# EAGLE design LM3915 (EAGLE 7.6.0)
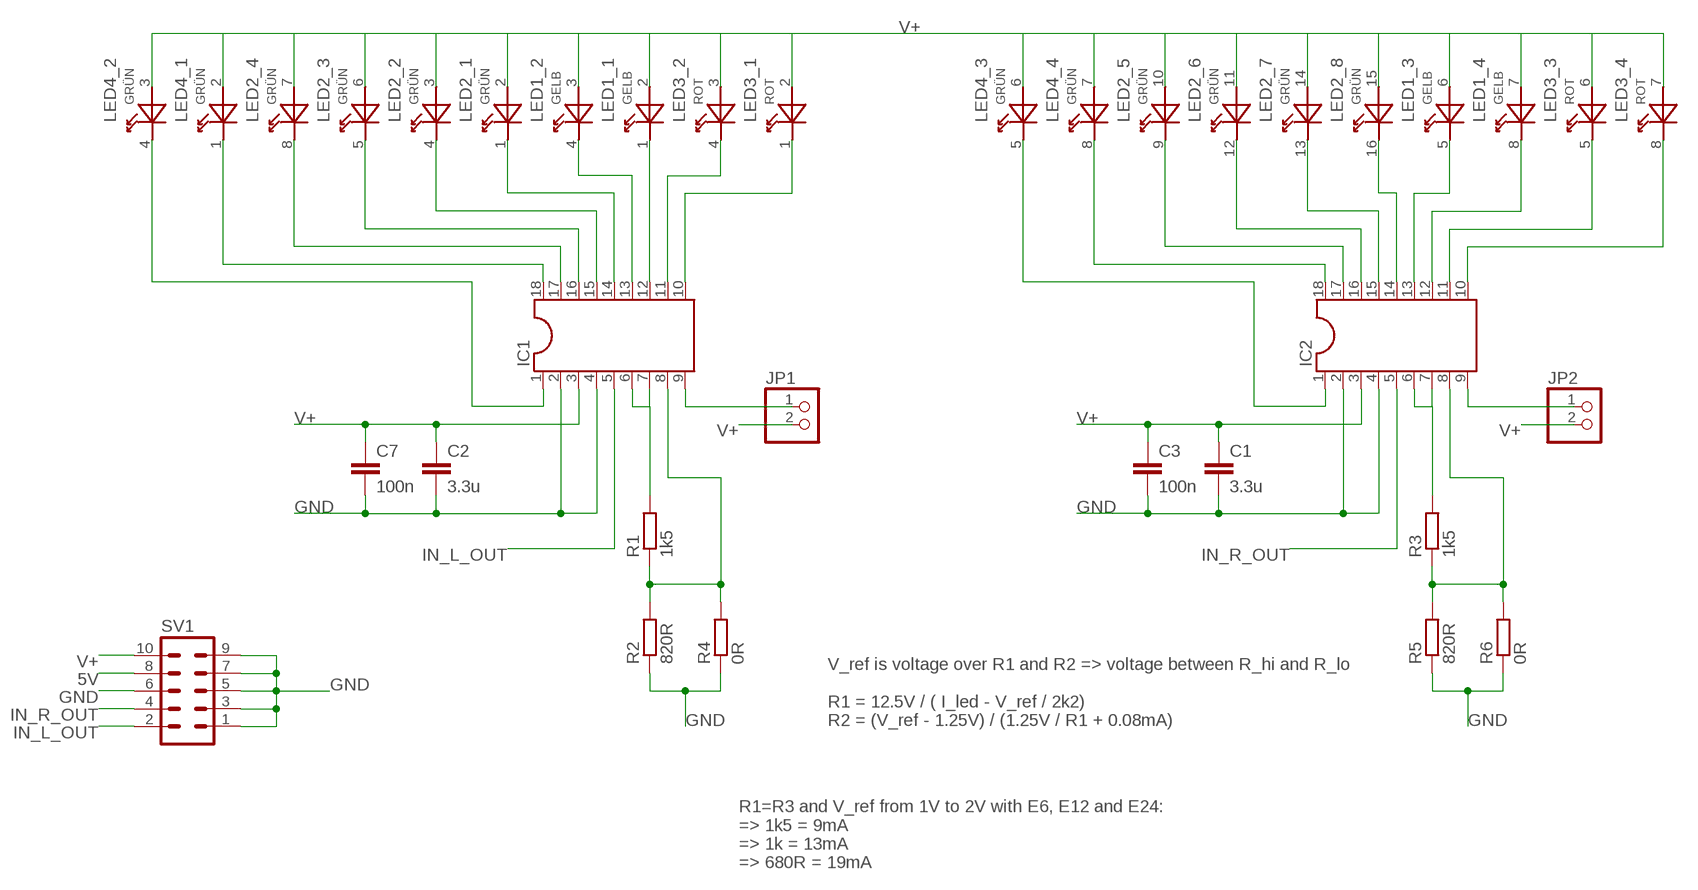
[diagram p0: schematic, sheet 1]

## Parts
C1  3.3u  C-EU050-055X075  [C050-055X075]
C2  3.3u  C-EU050-055X075  [C050-055X075]
C3  100n  C-EU050-025X075  [C050-025X075]
C7  100n  C-EU050-025X075  [C050-025X075]
IC1  DIL18S  [SOCKET-18]
IC2  DIL18S  [SOCKET-18]
JP1  PINHD-1X2  [1X02]
JP2  PINHD-1X2  [1X02]
LED1  GELB  KB-27XX-2  [KB-27XX]
LED2  GRÜN  KB-28XX-4  [KB-28XX]
LED3  ROT  KB-27XX-2  [KB-27XX]
LED4  GRÜN  KB-27XX-2  [KB-27XX]
R1  1k5  R-EU_0309/V  [0309V]
R2  820R  R-EU_0309/V  [0309V]
R3  1k5  R-EU_0309/V  [0309V]
R4  0R  R-EU_R0603  [R0603]
R5  820R  R-EU_0309/V  [0309V]
R6  0R  R-EU_R0603  [R0603]
SV1  ML10  [ML10]

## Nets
5V: SV1.8
GND: C1.2 C2.2 C3.2 C7.2 IC1.2 IC1.4 IC2.2 IC2.4 R2.1 R4.1 R5.1 R6.1 SV1.1 SV1.3 SV1.5 SV1.6 SV1.7 SV1.9
IN_L_OUT: IC1.5 SV1.2
IN_R_OUT: IC2.5 SV1.4
N$1: IC1.9 JP1.1
N$2: IC1.6 IC1.7 R1.2
N$3: IC1.8 R1.1 R2.2 R4.2
N$4: IC2.6 IC2.7 R3.2
N$5: IC2.9 JP2.1
N$6: IC2.8 R3.1 R5.2 R6.2
N$7: IC1.1 LED4.4(_2:P1)
N$8: IC1.18 LED4.1(_1:P1)
N$9: IC1.17 LED2.8(_4:P1)
N$10: IC1.16 LED2.5(_3:P1)
N$11: IC1.15 LED2.4(_2:P1)
N$12: IC1.14 LED2.1(_1:P1)
N$13: IC1.13 LED1.4(_2:P1)
N$14: IC1.12 LED1.1(_1:P1)
N$15: IC1.11 LED3.4(_2:P1)
N$16: IC1.10 LED3.1(_1:P1)
N$18: IC2.18 LED4.8(_4:P1)
N$19: IC2.17 LED2.9(_5:P1)
N$20: IC2.16 LED2.12(_6:P1)
N$21: IC2.15 LED2.13(_7:P1)
N$22: IC2.14 LED2.16(_8:P1)
N$23: IC2.13 LED1.5(_3:P1)
N$24: IC2.12 LED1.8(_4:P1)
N$25: IC2.11 LED3.5(_3:P1)
N$26: IC2.10 LED3.8(_4:P1)
N$27: IC2.1 LED4.5(_3:P1)
V+: C1.1 C2.1 C3.1 C7.1 IC1.3 IC2.3 JP1.2 JP2.2 LED1.2(_1:P2) LED1.3(_2:P2) LED1.6(_3:P2) LED1.7(_4:P2) LED2.2(_1:P2) LED2.3(_2:P2) LED2.6(_3:P2) LED2.7(_4:P2) LED2.10(_5:P2) LED2.11(_6:P2) LED2.14(_7:P2) LED2.15(_8:P2) LED3.2(_1:P2) LED3.3(_2:P2) LED3.6(_3:P2) LED3.7(_4:P2) LED4.2(_1:P2) LED4.3(_2:P2) LED4.6(_3:P2) LED4.7(_4:P2) SV1.10

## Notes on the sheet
- V_ref is voltage over R1 and R2 => voltage between R_hi and R_lo
  
  R1 = 12.5V / ( I_led - V_ref / 2k2)
  R2 = (V_ref - 1.25V) / (1.25V / R1 + 0.08mA)
- R1=R3 and V_ref from 1V to 2V with E6, E12 and E24:
  => 1k5 = 9mA 
  => 1k = 13mA
  => 680R = 19mA

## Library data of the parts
C1-C3 C7 = rcl:C-EU: CAPACITOR, European symbol
IC1 IC2 = ic-package:DIL18: Dual In Line / Socket
JP1 JP2 = pinhead:PINHD-1X2: PIN HEADER
LED1 LED3 LED4 = my:KB-27XX-2: FW-LED 10x10 GE reichelt.de
LED2 = my:KB-28XX-4: FW-LED 10X20 GN reichelt.de
R1-R6 = rcl:R-EU_: RESISTOR, European symbol
SV1 = con-ml:ML10: HARTING; OC_FARNELL: unknown; OC_NEWARK: unknown

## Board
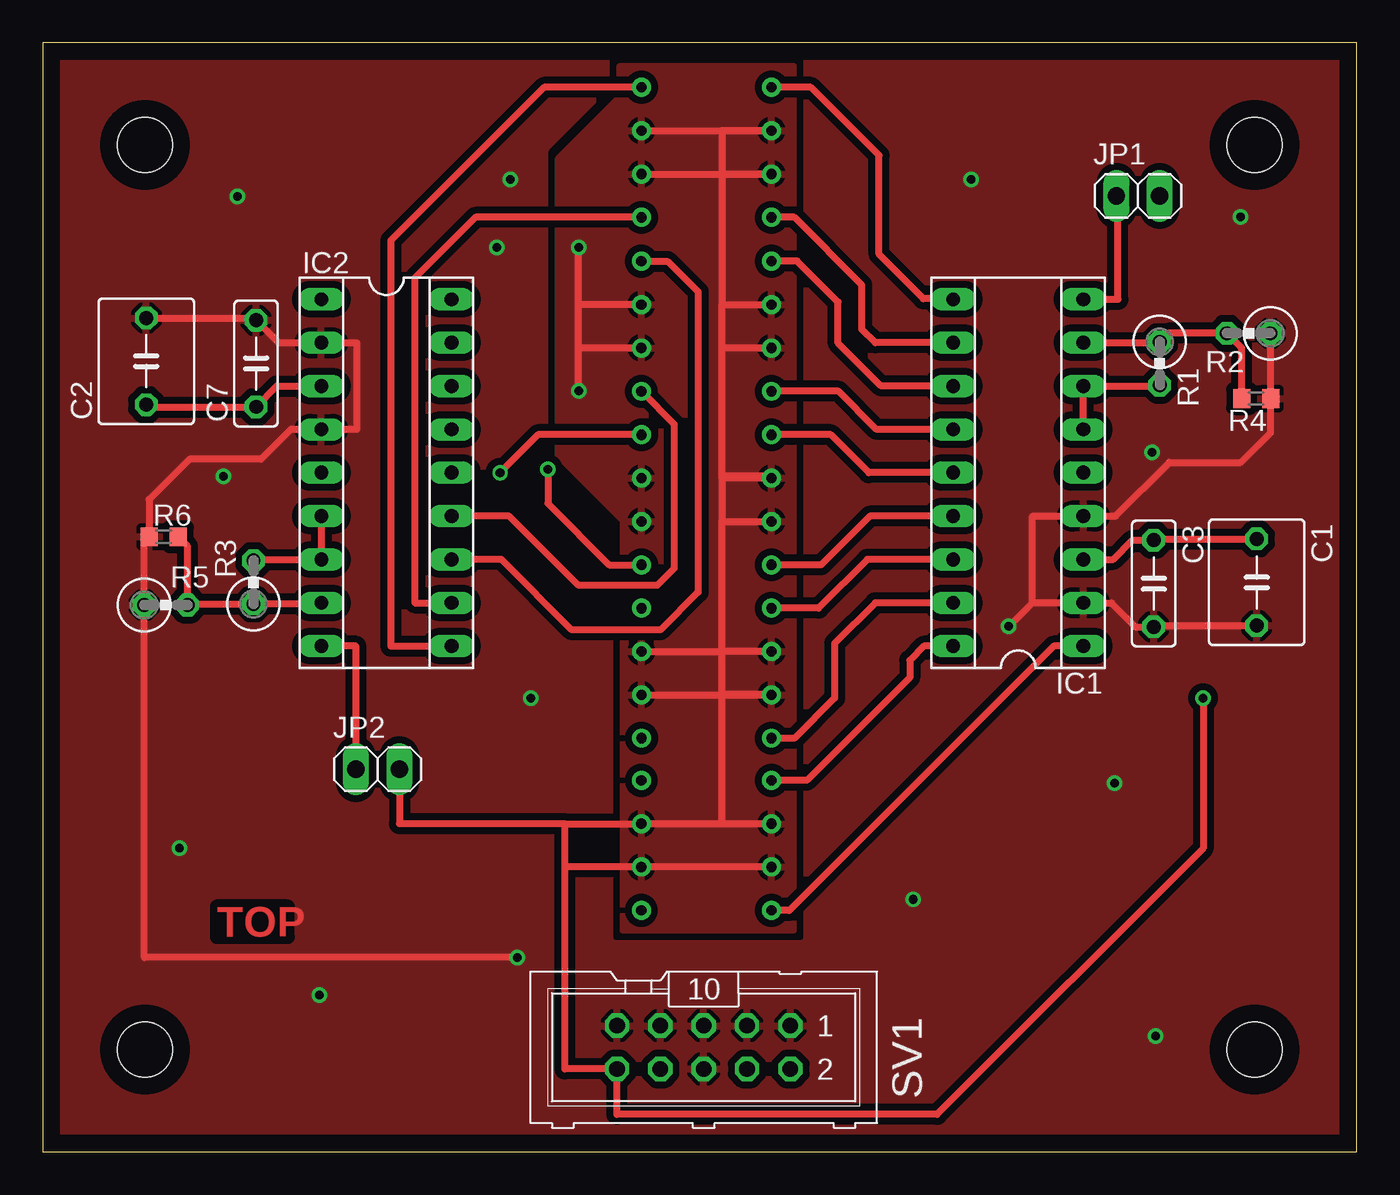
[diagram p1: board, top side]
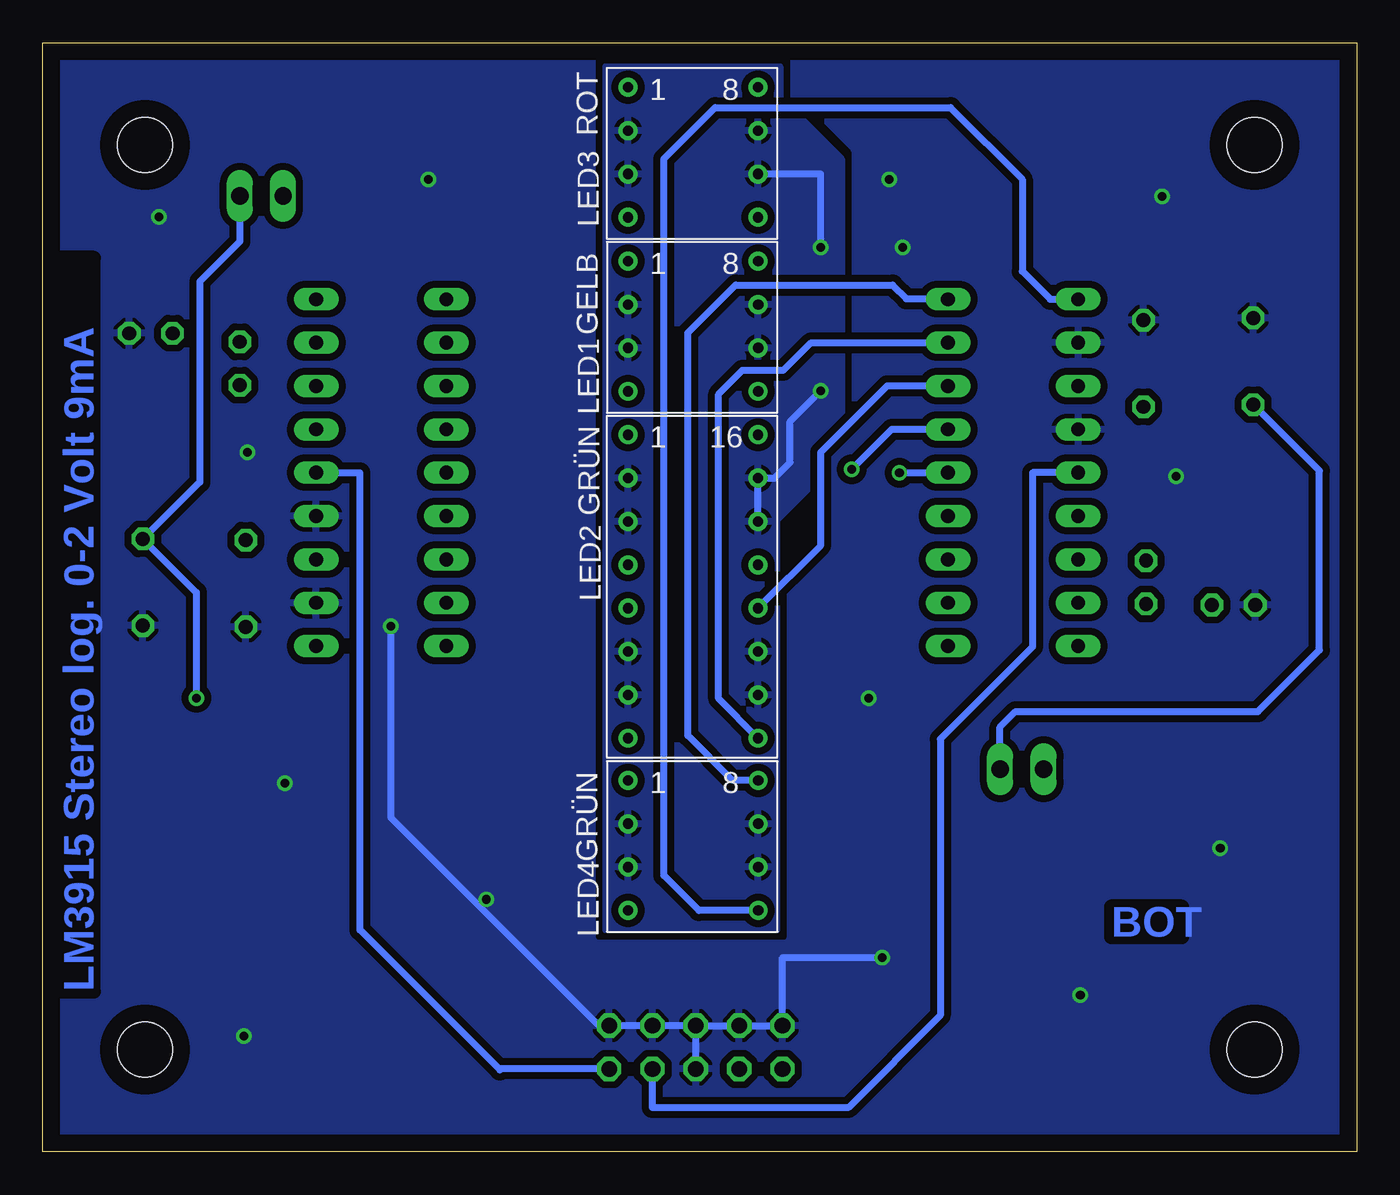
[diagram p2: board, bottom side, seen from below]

Size 77 x 65 mm. Coordinates in mm from the lower left corner, seen from the top.
Outline: 0,0 77,0 77,65 0,65 0,0
Copper layers (1*16): Top 0.035mm / dielectric 1.5mm / Bottom 0.035mm
Design rules "default *": minimum track width 10mil, minimum drill 0.5mm, track to track 8mil, track to pad 8mil, pad to pad 8mil, via to via 8mil, smd to smd 8mil, copper to edge 40mil, drill to drill 8mil, minimum pad ring 10mil, minimum via ring 8mil, stop-mask expansion 4mil, vias tented up to drill 0mil, thermal gap 10mil
Holes 3.2 mm at 6,59 6,6 71,59 71,6

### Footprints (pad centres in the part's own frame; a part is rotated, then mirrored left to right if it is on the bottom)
C050-055X075 = drill 0.813 octagon: 1 -2.54,0; 2 2.54,0
C050-025X075 = drill 0.813 octagon: 1 -2.54,0; 2 2.54,0
SOCKET-18 = drill 0.813 long: 1 -10.16,-3.81; 2 -7.62,-3.81; 3 -5.08,-3.81; 4 -2.54,-3.81; 5 0,-3.81; 6 2.54,-3.81; 7 5.08,-3.81; 8 7.62,-3.81; 9 10.16,-3.81; 10 10.16,3.81; 11 7.62,3.81; 12 5.08,3.81; 13 2.54,3.81; 14 0,3.81; 15 -2.54,3.81; 16 -5.08,3.81; 17 -7.62,3.81; 18 -10.16,3.81
1X02 = drill 1.016 long: 1 -1.27,0; 2 1.27,0
KB-27XX = drill 0.6: 1 0,0; 2 0,-2.54; 3 0,-5.08; 4 0,-7.62; 5 7.62,-7.62; 6 7.62,-5.08; 7 7.62,-2.54; 8 7.62,0
KB-28XX = drill 0.6: 1 0,0; 2 0,-2.54; 3 0,-5.08; 4 0,-7.62; 5 0,-10.16; 6 0,-12.7; 7 0,-15.24; 8 0,-17.78; 9 7.62,-17.78; 10 7.62,-15.24; 11 7.62,-12.7; 12 7.62,-10.16; 13 7.62,-7.62; 14 7.62,-5.08; 15 7.62,-2.54; 16 7.62,0
0309V = drill 0.813 octagon: 1 -1.27,0; 2 1.27,0
R0603 = smd 1 x 1.1: 1 -0.85,0; 2 0.85,0
ML10 = drill 0.914 octagon: 1 -5.08,-1.27; 2 -5.08,1.27; 3 -2.54,-1.27; 4 -2.54,1.27; 5 0,-1.27; 6 0,1.27; 7 2.54,-1.27; 8 2.54,1.27; 9 5.08,-1.27; 10 5.08,1.27

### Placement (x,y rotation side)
C1  71.13,33.38 270 top
C2  6.07,46.33 90 top
C3  65.1,33.31 270 top
C7  12.5,46.2 90 top
IC1  57.16,39.8 90 top
IC2  20.14,39.8 270 top
JP1  64.18,56.03 0 top
JP2  19.63,22.43 0 top
LED1  42.7,52.19 0 bottom
LED2  42.7,42.02 0 bottom
LED3  42.7,62.38 0 bottom
LED4  42.7,21.77 0 bottom
R1  65.45,46.2 270 top
R2  70.66,47.97 180 top
R3  12.35,33.38 90 top
R4  71.1,44.15 180 top
R5  7.22,32.05 0 top
R6  7.09,36.05 0 top
SV1  38.73,6.13 180 top

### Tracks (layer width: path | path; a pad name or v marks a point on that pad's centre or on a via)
GND  (via drill 0.5)
  Top 0.406: C2.2 12.5,48.87 C7.2 13.82,47.42 IC2.2 18.4,47.42 18.4,42.34 IC2.4 14.54,42.34 12.8,40.6 8.6,40.6 6.24,38.24 R6.1 5.95,35.76 R5.1 5.95,11.4 v27.8,11.4 | R2.1 71.93,44.17 R4.1 71.95,42.15 70.2,40.4 66,40.4 62.86,37.26 IC1.4 58,37.26 58,32.18 | C1.2 65.17,30.84 C3.2 64.03,30.77 62.62,32.18 IC1.2 58,32.18 | 58,32.18 56.62,30.8 v56.6,30.8
  Bottom 0.406: SV1.6 SV1.5 | SV1.5 SV1.7 SV1.9 33.65,11.4 v27.8,11.4 | SV1.5 SV1.3 SV1.1 44.4,7.4 56.6,19.6 v56.6,30.8
  other vias: 11.4,56 10.6,39.6 8,17.8 16.2,9.2 51,14.8 62.8,21.6 65.2,6.8 65,41 70.2,54.8 54.4,57 27.4,57 26.6,53 28.6,26.6
  pour Top (isolate 0.406, rank 2): 0.2,64.8 76.8,64.8 76.8,0.2 0.2,0.2
  pour Bottom (isolate 0.406, rank 2): 0.2,64.8 76.8,64.8 76.8,0.2 0.2,0.2
IN_L_OUT
  Bottom 0.406: IC1.5 58.4,39.8 58.4,13 50.2,4.8 50.2,4.86 SV1.2
IN_R_OUT
  Bottom 0.406: IC2.5 19,39.8 19,29.6 24.4,24.2 24.4,8 29.8,2.6 41.27,2.6 SV1.4
N$1
  Top 0.406: IC1.9 63,49.96 63,56.06 JP1.1
N$2
  Top 0.406: R1.2 65.4,44.88 IC1.7 IC1.6
N$3
  Top 0.406: IC1.8 65.4,47.42 R1.1 65.95,47.97 R2.2 70.25,47.11 R4.2
N$4
  Top 0.406: R3.2 12.42,34.72 IC2.7 IC2.6
N$5
  Top 0.406: JP2.1 18.36,29.64 IC2.9
N$6
  Top 0.406: IC2.8 16.26,32.11 R3.1 8.55,32.11 R5.2 8.49,35.5 R6.2
N$7
  Top 0.406: IC1.1 59.24,29.64 43.75,14.15 LED4.4
N$8
  Top 0.406: IC1.18 51.64,29.64 50.8,28.8 50.8,27.8 44.77,21.77 LED4.1
N$9
  Top 0.406: IC1.17 48.78,32.18 46.4,29.8 46.4,26.6 44.04,24.24 LED2.8
N$10
  Top 0.406: IC1.16 48.32,34.72 45.46,31.86 LED2.5
N$11
  Top 0.406: IC1.15 48.46,37.26 45.6,34.4 LED2.4
N$12
  Top 0.406: IC1.14 48.4,39.8 46.18,42.02 LED2.1
N$13
  Top 0.406: IC1.13 48.86,42.34 46.63,44.57 LED1.4
N$14
  Top 0.406: IC1.12 49.12,44.88 46.6,47.4 46.6,49.8 44.2,52.2 LED1.1
N$15
  Top 0.406: IC1.11 48.78,47.42 48,48.2 48,50.8 44.03,54.77 LED3.4
N$16
  Top 0.406: IC1.10 53.31,50 51.6,50 49,52.6 49,58.4 45.02,62.38 LED3.1
N$18
  Bottom 0.406: LED4.8 36.57,21.77 39.2,24.4 39.2,48 36.4,50.8 27.2,50.8 26.4,50 23.99,50 IC2.18
N$19
  Bottom 0.406: LED2.9 37.4,26.56 37.4,44.4 36,45.8 33.6,45.8 31.98,47.42 IC2.17
N$20
  Bottom 0.406: LED2.12 31.4,35.55 31.4,41 27.52,44.88 IC2.16
N$21  (via drill 0.5)
  Top 0.406: v29.6,40 29.6,38 33.2,34.4 LED2.13
  Bottom 0.406: IC2.15 27.26,42.34 v29.6,40
N$22  (via drill 0.5)
  Top 0.406: LED2.16 29.02,42.02 v26.8,39.8
  Bottom 0.406: v26.8,39.8 IC2.14
N$23
  Top 0.406: LED1.5 37,42.65 37,34.2 36,33.2 31.4,33.2 27.34,37.26 IC2.13
N$24
  Top 0.406: LED1.8 36.61,52.19 38.4,50.4 38.4,32.8 36.2,30.6 31,30.6 26.88,34.72 IC2.12
N$25
  Top 0.406: LED3.5 25.36,54.77 21.8,51.2 21.8,32.18 IC2.11
N$26
  Top 0.406: LED3.8 29.39,62.38 20.4,53.4 20.4,29.64 21.8,29.64 22,29.64 IC2.10
N$27
  Bottom 0.406: LED4.5 38.55,14.15 40.6,16.2 40.6,58.2 37.6,61.2 23.8,61.2 19.6,57 19.6,51.6 17.96,49.96 IC2.1
V+  (via drill 0.5)
  Top 0.406: IC2.3 13.72,44.88 C7.1 6.2,43.66 C2.1 | 30.6,16.69 30.6,4.86 SV1.10 33.65,2.2 52.4,2.2 68,17.8 v68,26.6 | 30.6,16.69 30.6,19.23 | 30.6,19.23 LED4.7 LED4.2 39.8,19.23 39.8,26.8 | 30.6,16.69 LED4.6 LED4.3 | 30.6,19.23 20.9,19.23 JP2.2 | C1.1 65.17,35.92 C3.1 63.85,35.85 62.72,34.72 IC1.3 | LED2.10 LED2.7 42.7,26.8 39.8,26.8 | LED2.11 39.8,29.32 | 39.8,26.8 39.8,29.32 | LED2.6 39.8,29.32 | 39.8,29.32 39.8,36 39.8,36.94 | 39.8,36.94 LED2.3 | 39.8,47.11 39.8,39.6 42.7,39.6 LED2.2 39.8,39.48 39.8,36.94 | 39.8,47.11 39.8,49.65 | 39.8,49.65 LED1.2 | LED1.6 31.4,47.11 | 31.4,47.11 31.4,49.65 | 31.4,49.65 v31.4,53 | LED3.7 LED3.2 39.8,59.84 39.8,57.3 | LED3.6 LED3.3 39.8,57.3 | 39.8,57.3 39.8,49.65 | LED1.7 31.4,49.65 | LED1.3 39.8,47.11 | v31.4,44.6 31.4,47.11
  Bottom 0.406: JP2.2 20.9,24.9 20,25.8 5.8,25.8 2.2,29.4 2.2,39.92 C2.1 | v68,26.6 68,32.79 C1.1 67.8,39.25 67.8,51 65.45,53.35 JP1.2 | v31.4,53 31.4,57.3 LED3.6 | LED2.14 LED2.15 34.12,39.48 33.2,40.4 33.2,42.8 v31.4,44.6
  pour Top (isolate 0.406): 33.8,63.6 33.8,61.8 30.2,58.2 30.2,40.8 34,37 34,13 44,13 44,63.6
  pour Bottom (isolate 0.406): 33.8,63.6 33.8,61.8 30.2,58.2 30.2,40.8 34,37 34,13 44,13 44,63.6

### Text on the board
Top: TOP
Bottom: BOT | LM3915 Stereo log. 0-2 Volt 9mA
